| TEXAS INSTRUMENTS INCORPORATED
| Standard Linear and Logic Group
| IBIS Model of SN74LVCH244A
| OCTAL BUFFERS/DRIVERS WITH 3-STATE OUTPUTS
| This file contains package information for the following:
|  SOIC 20-pin (DW) package as [Component] LVCH244A_DW
|  SSOP 20-pin (DB) package as [Component] LVCH244A_DB
|  TSSOP 20-pin (PW) package as [Component] LVCH244A_PW
|  TVSOP 20-pin (DGV) package as [Component] LVCH244A_DGV
|  SOP 20-pin (NS) package as [Component] LVCH244A_NS
| This device can be powered at the following Vccs:
|  1.8 volt Vcc
|  2.5 volt Vcc
|  3.3 volt Vcc
| This file provides unique models under the [Model Selector] for each Vcc.
| For operation at a specific Vcc, select the appropriate model after each
| [Model Selector] keyword.
[IBIS Ver]   3.2
[Comment char]  |_char
[File Name]   sn74lvch244a.ibs
[File Rev]   1.1 | e_die
[Date]   April 25, 2002
[Source]   Data created from TI-SPICE simulations at TI-SLL.
[Notes]   The following is an IBIS list for the SN74LVCH244A.
   Please contact sllibis@ti.com with questions and
   comments concerning SLL IBIS models.
   This IBIS model is created from a BA (back annotated netlist).
   - Non-monotonic data in ground-clamp due to bus hold.
   - Due to the fact that the device is 5-V input/output
   tolerant, the output model has some non-monotonic
   warnings.
[Disclaimer] Property of Texas Instruments Incorporated.  Unauthorized
   reproduction and/or distribution is strictly prohibited.
   This product is protected under copyright law.
   Created  2002, (C) Copyright  2002, Texas Instruments
   Incorporated, All Rights Reserved
   UNLESS THERE IS A SIGNED, WRITTEN AGREEMENT TO THE
   CONTRARY, TEXAS INSTRUMENTS (TI) IS PROVIDING THE IBIS
   MODELS  AND WITHOUT ANY WARRANTY, EXPRESSED OR
   IMPLIED.  TI assumes no liability for:
   1) the accuracy of the IBIS models provided to your
   company;
   2) the proper functioning of these IBIS Models in your
   design or for any resulting applications; or
   3) infringement of patents, copyrights or intellectual
   property rights resulting from your use of these IBIS
   models.
   TI provides IBIS Models as a service to our customers.
   You and your company shall not distribute, sell or give
   these models to anyone else without prior written
   permission from TI.
   TI reserves the right to make changes to our products or
   to discontinue any semiconductor product or service
   without notice, and advises our customers to obtain the
   latest version of relevant information to verify, before
   placing orders, that the information being relied on is
   current.
   Please be aware that your receipt and use of the IBIS
   information provided shall serve as acceptance of these
   terms and conditions.  If you do not accept these terms,
   you should return or destroy the IBIS models and any
   other accompanying information immediately.
| Component LVCH244A_DW 20-pin SOIC
[Component]   LVCH244A_DW
[Manufacturer]  Texas Instruments, Inc.
[Package]
|   typ   min   max
R_pkg   3.800e-02   3.300e-02   4.500e-02
L_pkg   5.012e-09   4.110e-09   6.349e-09
C_pkg   7.170e-13   5.300e-13   8.680e-13
[Pin]   signal_name   model_name   R_pin   L_pin   C_pin
1   1NOE   LVCH244A_NOE   4.200e-02   6.336e-09   8.650e-13
2   1A1   LVCH244A_IN   4.300e-02   5.542e-09   8.670e-13
3   2Y4   LVCH244A_OUT   3.400e-02   4.714e-09   7.320e-13
4   1A2   LVCH244A_IN   3.400e-02   4.377e-09   5.910e-13
5   2Y3   LVCH244A_OUT   3.600e-02   4.130e-09   5.330e-13
6   1A3   LVCH244A_IN   3.500e-02   4.111e-09   5.300e-13
7   2Y2   LVCH244A_OUT   3.400e-02   4.284e-09   5.830e-13
8   1A4   LVCH244A_IN   3.400e-02   4.634e-09   7.260e-13
9   2Y1   LVCH244A_OUT   4.000e-02   5.518e-09   8.650e-13
10   GND   GND   4.300e-02   6.349e-09   8.660e-13
11   2A1   LVCH244A_IN   4.100e-02   6.281e-09   8.610e-13
12   1Y4   LVCH244A_OUT   4.500e-02   5.561e-09   8.680e-13
13   2A2   LVCH244A_IN   3.300e-02   4.778e-09   7.420e-13
14   1Y3   LVCH244A_OUT   3.500e-02   4.414e-09   5.960e-13
15   2A3   LVCH244A_IN   3.500e-02   4.110e-09   5.330e-13
16   1Y2   LVCH244A_OUT   3.600e-02   4.130e-09   5.330e-13
17   2A4   LVCH244A_IN   3.400e-02   4.377e-09   5.910e-13
18   1Y1   LVCH244A_OUT   3.400e-02   4.714e-09   7.310e-13
19   2NOE   LVCH244A_NOE   4.300e-02   5.569e-09   8.680e-13
20   VCC   POWER   4.200e-02   6.308e-09   8.640e-13
| Component LVCH244A_DB 20-pin SSOP
[Component]   LVCH244A_DB
[Manufacturer]  Texas Instruments, Inc.
[Package]
|   typ   min   max
R_pkg   4.000e-02   3.500e-02   5.100e-02
L_pkg   3.495e-09   3.035e-09   4.314e-09
C_pkg   4.200e-13   3.460e-13   5.020e-13
[Pin]   signal_name   model_name   R_pin   L_pin   C_pin
1   1NOE   LVCH244A_NOE   4.900e-02   4.310e-09   5.020e-13
2   1A1   LVCH244A_IN   4.800e-02   3.903e-09   4.870e-13
3   2Y4   LVCH244A_OUT   3.500e-02   3.189e-09   3.960e-13
4   1A2   LVCH244A_IN   3.500e-02   3.036e-09   3.470e-13
5   2Y3   LVCH244A_OUT   3.500e-02   3.035e-09   3.670e-13
6   1A3   LVCH244A_IN   3.500e-02   3.035e-09   3.670e-13
7   2Y2   LVCH244A_OUT   3.500e-02   3.036e-09   3.470e-13
8   1A4   LVCH244A_IN   3.500e-02   3.189e-09   3.970e-13
9   2Y1   LVCH244A_OUT   4.700e-02   3.899e-09   4.880e-13
10   GND   GND   5.100e-02   4.314e-09   5.000e-13
11   2A1   LVCH244A_IN   5.100e-02   4.314e-09   5.000e-13
12   1Y4   LVCH244A_OUT   4.700e-02   3.899e-09   4.880e-13
13   2A2   LVCH244A_IN   3.500e-02   3.189e-09   3.970e-13
14   1Y3   LVCH244A_OUT   3.500e-02   3.036e-09   3.460e-13
15   2A3   LVCH244A_IN   3.500e-02   3.035e-09   3.670e-13
16   1Y2   LVCH244A_OUT   3.500e-02   3.035e-09   3.670e-13
17   2A4   LVCH244A_IN   3.500e-02   3.036e-09   3.460e-13
18   1Y1   LVCH244A_OUT   3.500e-02   3.189e-09   3.970e-13
19   2NOE   LVCH244A_NOE   4.700e-02   3.899e-09   4.880e-13
20   VCC   POWER   5.100e-02   4.314e-09   5.020e-13
| Component LVCH244A_PW 20-pin TSSOP
[Component]   LVCH244A_PW
[Manufacturer]  Texas Instruments, Inc.
[Package]
|   typ   min   max
R_pkg   5.000e-02   4.200e-02   6.000e-02
L_pkg   2.802e-09   2.248e-09   3.553e-09
C_pkg   3.170e-13   2.020e-13   4.430e-13
[Pin]   signal_name   model_name   R_pin   L_pin   C_pin
1   1NOE   LVCH244A_NOE   5.500e-02   3.461e-09   4.400e-13
2   1A1   LVCH244A_IN   5.500e-02   3.150e-09   4.010e-13
3   2Y4   LVCH244A_OUT   4.200e-02   2.619e-09   3.020e-13
4   1A2   LVCH244A_IN   4.500e-02   2.273e-09   2.020e-13
5   2Y3   LVCH244A_OUT   4.500e-02   2.248e-09   2.240e-13
6   1A3   LVCH244A_IN   4.500e-02   2.273e-09   2.260e-13
7   2Y2   LVCH244A_OUT   4.400e-02   2.323e-09   2.050e-13
8   1A4   LVCH244A_IN   4.600e-02   2.704e-09   3.070e-13
9   2Y1   LVCH244A_OUT   6.000e-02   3.265e-09   4.110e-13
10   GND   GND   5.700e-02   3.506e-09   4.360e-13
11   2A1   LVCH244A_IN   5.800e-02   3.553e-09   4.370e-13
12   1Y4   LVCH244A_OUT   5.800e-02   3.193e-09   4.050e-13
13   2A2   LVCH244A_IN   4.200e-02   2.704e-09   3.110e-13
14   1Y3   LVCH244A_OUT   4.600e-02   2.392e-09   2.100e-13
15   2A3   LVCH244A_IN   4.700e-02   2.334e-09   2.290e-13
16   1Y2   LVCH244A_OUT   4.700e-02   2.300e-09   2.270e-13
17   2A4   LVCH244A_IN   4.700e-02   2.349e-09   2.070e-13
18   1Y1   LVCH244A_OUT   4.500e-02   2.677e-09   3.060e-13
19   2NOE   LVCH244A_NOE   6.000e-02   3.235e-09   4.060e-13
20   VCC   POWER   5.600e-02   3.487e-09   4.430e-13
| Component LVCH244A_DGV 20-pin TVSOP
[Component]   LVCH244A_DGV
[Manufacturer]  Texas Instruments, Inc.
[Package]
|   typ   min   max
R_pkg   4.400e-02   3.800e-02   4.800e-02
L_pkg   2.561e-09   2.236e-09   2.961e-09
C_pkg   3.420e-13   2.640e-13   4.460e-13
[Pin]   signal_name   model_name   R_pin   L_pin   C_pin
1   1NOE   LVCH244A_NOE   4.400e-02   2.935e-09   4.170e-13
2   1A1   LVCH244A_IN   4.200e-02   2.869e-09   4.460e-13
3   2Y4   LVCH244A_OUT   4.300e-02   2.399e-09   3.160e-13
4   1A2   LVCH244A_IN   4.400e-02   2.236e-09   2.650e-13
5   2Y3   LVCH244A_OUT   4.600e-02   2.278e-09   2.640e-13
6   1A3   LVCH244A_IN   4.500e-02   2.274e-09   2.640e-13
7   2Y2   LVCH244A_OUT   4.400e-02   2.285e-09   2.690e-13
8   1A4   LVCH244A_IN   4.300e-02   2.452e-09   3.200e-13
9   2Y1   LVCH244A_OUT   4.400e-02   2.900e-09   4.460e-13
10   GND   GND   4.400e-02   2.961e-09   4.180e-13
11   2A1   LVCH244A_IN   4.500e-02   2.954e-09   4.180e-13
12   1Y4   LVCH244A_OUT   4.200e-02   2.847e-09   4.430e-13
13   2A2   LVCH244A_IN   4.500e-02   2.453e-09   3.190e-13
14   1Y3   LVCH244A_OUT   4.500e-02   2.297e-09   2.690e-13
15   2A3   LVCH244A_IN   4.800e-02   2.334e-09   2.680e-13
16   1Y2   LVCH244A_OUT   4.800e-02   2.335e-09   2.670e-13
17   2A4   LVCH244A_IN   4.600e-02   2.299e-09   2.680e-13
18   1Y1   LVCH244A_OUT   4.600e-02   2.457e-09   3.200e-13
19   2NOE   LVCH244A_NOE   4.300e-02   2.848e-09   4.410e-13
20   VCC   POWER   3.800e-02   2.812e-09   4.080e-13
| Component LVCH244A_NS 20-pin SOP
[Component]   LVCH244A_NS
[Manufacturer]  Texas Instruments, Inc.
[Package]
|   typ   min   max
R_pkg   4.400e-02   2.900e-02   5.800e-02
L_pkg   3.666e-09   2.317e-09   5.115e-09
C_pkg   5.480e-13   3.160e-13   7.250e-13
[Pin]   signal_name   model_name   R_pin   L_pin   C_pin
1   1NOE   LVCH244A_NOE   5.800e-02   5.115e-09   7.250e-13
2   1A1   LVCH244A_IN   5.300e-02   4.591e-09   7.240e-13
3   2Y4   LVCH244A_OUT   4.900e-02   3.754e-09   5.720e-13
4   1A2   LVCH244A_IN   2.900e-02   2.549e-09   3.880e-13
5   2Y3   LVCH244A_OUT   3.100e-02   2.317e-09   3.160e-13
6   1A3   LVCH244A_IN   3.100e-02   2.317e-09   3.160e-13
7   2Y2   LVCH244A_OUT   2.900e-02   2.556e-09   3.990e-13
8   1A4   LVCH244A_IN   4.900e-02   3.754e-09   5.790e-13
9   2Y1   LVCH244A_OUT   5.300e-02   4.591e-09   7.240e-13
10   GND   GND   5.800e-02   5.115e-09   7.250e-13
11   2A1   LVCH244A_IN   5.800e-02   5.115e-09   7.250e-13
12   1Y4   LVCH244A_OUT   5.300e-02   4.591e-09   7.240e-13
13   2A2   LVCH244A_IN   4.900e-02   3.754e-09   5.790e-13
14   1Y3   LVCH244A_OUT   2.900e-02   2.557e-09   3.990e-13
15   2A3   LVCH244A_IN   3.100e-02   2.317e-09   3.160e-13
16   1Y2   LVCH244A_OUT   3.100e-02   2.317e-09   3.160e-13
17   2A4   LVCH244A_IN   2.900e-02   2.557e-09   3.990e-13
18   1Y1   LVCH244A_OUT   4.900e-02   3.754e-09   5.790e-13
19   2NOE   LVCH244A_NOE   5.300e-02   4.591e-09   7.240e-13
20   VCC   POWER   5.800e-02   5.115e-09   7.250e-13
| Model LVCH244A_NOE
[Model Selector]   LVCH244A_NOE
LVCH244A_NOE_18   1.8 volt Vcc
LVCH244A_NOE_25   2.5 volt Vcc
LVCH244A_NOE_33   3.3 volt Vcc
| Model LVCH244A_IN
[Model Selector]   LVCH244A_IN
LVCH244A_IN_18   1.8 volt Vcc
LVCH244A_IN_25   2.5 volt Vcc
LVCH244A_IN_33   3.3 volt Vcc
| Model LVCH244A_OUT
[Model Selector]   LVCH244A_OUT
LVCH244A_OUT_18   1.8 volt Vcc
LVCH244A_OUT_25   2.5 volt Vcc
LVCH244A_OUT_33   3.3 volt Vcc
| Models and submodels in the file (9): LVCH244A_NOE_18 (Input), LVCH244A_NOE_25 (Input), LVCH244A_NOE_33 (Input), LVCH244A_IN_18 (Input), LVCH244A_IN_25 (Input), LVCH244A_IN_33 (Input), LVCH244A_OUT_18 (3-state), LVCH244A_OUT_25 (3-state), LVCH244A_OUT_33 (3-state)
